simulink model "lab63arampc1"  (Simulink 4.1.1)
settings: Solver=ode45  StartTime=0.0  StopTime=10.0  MaxStep=.01  RelTol=1e-6
libraries: simulink3 x1

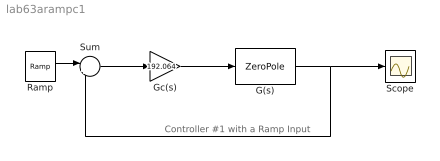
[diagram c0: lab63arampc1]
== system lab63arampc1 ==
  note: Controller #1 with a Ramp Input
  G(s) : ZeroPole  Zeros=[]  Poles=[0 -6 -10]  Gain=[1]  AbsoluteTolerance=auto
  Gc(s) : Gain  Gain=192.064  Multiplication=Element-wise(K.*u)  SaturateOnIntegerOverflow=on
  Ramp : simulink3/Sources/Ramp  slope=1  start=0  X0=0
  Scope : Scope
  Sum : Sum  Inputs=|+-  SaturateOnIntegerOverflow=on
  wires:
  Gc(s)/1 -> G(s)/1
  G(s)/1 -> Scope/1, Sum/2
  Sum/1 -> Gc(s)/1
  Ramp/1 -> Sum/1
